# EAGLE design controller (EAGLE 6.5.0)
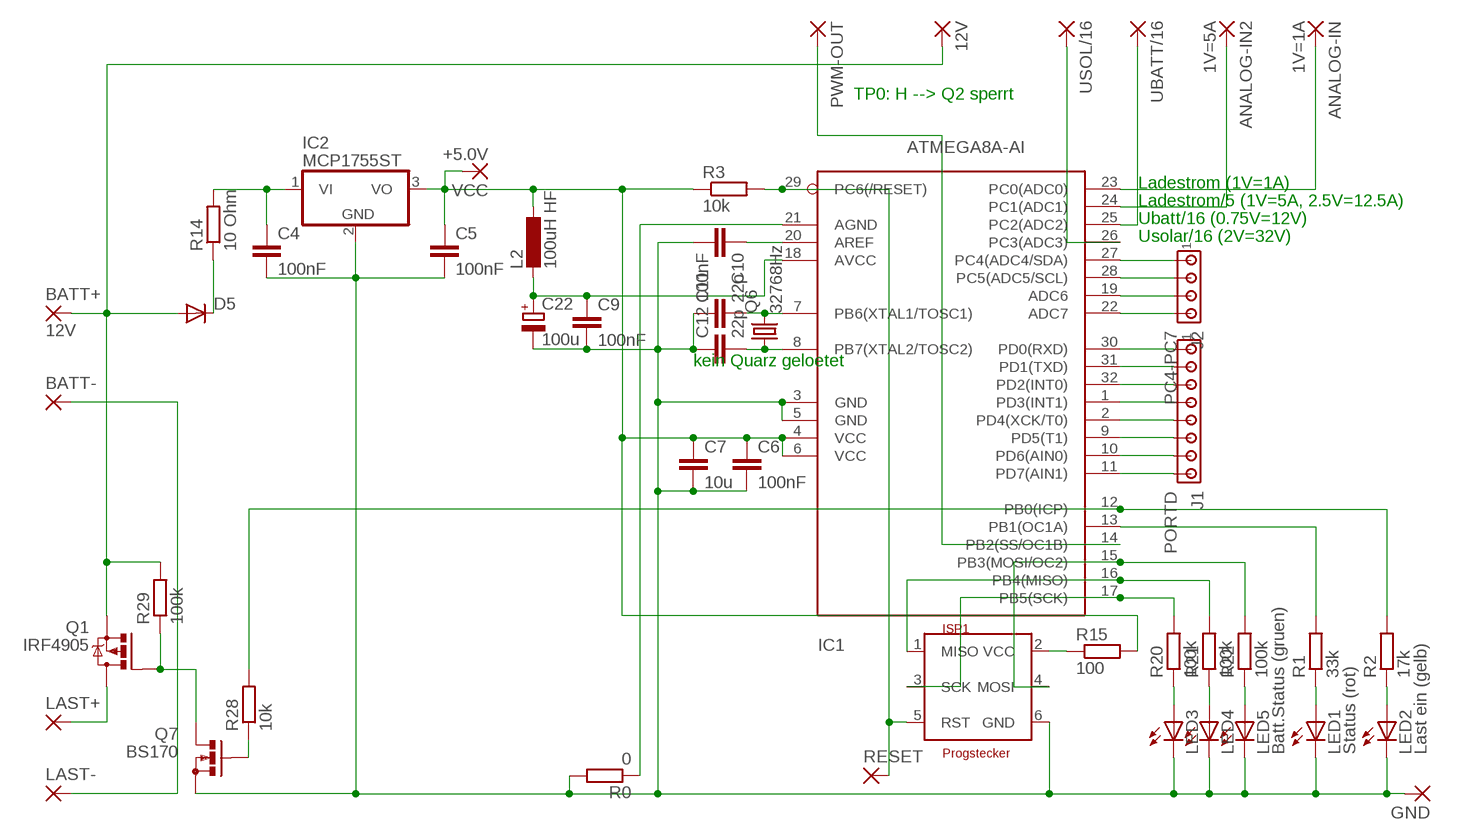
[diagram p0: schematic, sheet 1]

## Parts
12V  WIREPAD2,15/1,0  [2,15/1,0]
ANALOG-IN  1V=1A  WIREPAD2,15/1,0  [2,15/1,0]
ANALOG-IN2  1V=5A  WIREPAD2,15/1,0  [2,15/1,0]
BATT+  12V  WIREPAD3,81/1,1  [3,81/1,1]
BATT-  WIREPAD3,81/1,1  [3,81/1,1]
C4  100nF  C-EUC1206  [C1206]
C5  100nF  C-EUC1206  [C1206]
C6  100nF  C-EUC1206K  [C1206K]
C7  10u  C-EUC1206  [C1206]
C9  100nF  C-EUC1206K  [C1206K]
C10  100nF  C-EUC1206K  [C1206K]
C11  22p  C-EU025-024X044  [C025-024X044]
C12  22p  C-EU025-024X044  [C025-024X044]
C22  100u  CPOL-EUE2.5-5  [E2,5-5]
D5  1N4004  [DO41-10]
GND  WIREPAD2,15/1,0  [2,15/1,0]
IC1  ATMEGA8A-AI  MEGA8-AI  [TQFP32-08]
IC2  MCP1755ST  MCP1703DB  [SOT223]
ISP1  Progstecker  ISP6N  [ISP6]
J1  PORTD  MTA08-100  [10X08MTA]
J2  PC4-PC7  MTA04-100  [10X04MTA]
L2  100uH HF  L-EU0204/7  [0204/7]
LAST+  WIREPAD3,81/1,1  [3,81/1,1]
LAST-  WIREPAD3,81/1,1  [3,81/1,1]
LED1  Status (rot)  LEDSFH482  [SFH482]
LED2  Last ein (gelb)  LEDSFH482  [SFH482]
LED3  LEDSFH482  [SFH482]
LED4  LEDSFH482  [SFH482]
LED5  Batt.Status (gruen)  LEDSFH482  [SFH482]
PWM-OUT  WIREPAD2,15/1,0  [2,15/1,0]
Q1  IRF4905  IRF9530  [TO220BV]
Q6  32768Hz  CRYSTALTC26V  [TC26V]
Q7  BS170  [SOT54E]
R0  0  R-EU_R1206  [R1206]
R1  33k  R-EU_0204/2V  [0204V@1]
R2  17k  R-EU_0204/2V  [0204V@1]
R3  10k  R-EU_M1406  [M1406]
R14  10 Ohm  R-EU_0204/5  [0204/5@1]
R15  100  R-EU_0204/5  [0204/5@1]
R20  100k  R-EU_0204/2V  [0204V@1]
R21  100k  R-EU_0204/2V  [0204V@1]
R22  100k  R-EU_0204/2V  [0204V@1]
R28  10k  R-EU_0204/7  [0204/7@1]
R29  100k  R-EU_0204/5  [0204/5@1]
RESET  WIREPAD1,6/0,8  [1,6/0,8]
UBATT/16  WIREPAD2,15/1,0  [2,15/1,0]
USOL/16  WIREPAD2,15/1,0  [2,15/1,0]
VCC  +5.0V  WIREPAD2,54/0,9  [2,54/0,9]

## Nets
AGND [duenn]: IC1.21(AGND) R0.1
AVCC [duenn]: C9.1 C22.+ IC1.18(AVCC) L2.2
GND [dick]: C4.2 C5.2 C6.2 C7.2 C9.2 C10.2 C11.1 C12.1 C22.- GND.1(P) IC1.3(GND) IC1.5(GND) IC2.2(GND) ISP1.6(GND) LED1.K(C) LED2.K(C) LED3.K(C) LED4.K(C) LED5.K(C) Q7.S R0.2
N$1 [dick]: LED1.A R1.1
N$2: IC1.12(PB0(ICP)) R2.2 R28.2
N$3: IC1.17(PB5(SCK)) ISP1.3(SCK) R20.2
N$4: IC1.13(PB1(OC1A)) R1.2
N$5 [dick]: LED2.A R2.1
N$6 [duenn]: IC1.26(PC3(ADC3)) USOL/16.1(P)
N$7: IC1.14(PB2(SS/OC1B)) PWM-OUT.1(P)
N$8 [dick]: Q7.G R28.1
N$9 [duenn]: IC1.25(PC2(ADC2)) UBATT/16.1(P)
N$10: C10.1 IC1.20(AREF)
N$11: ISP1.2(VCC) R15.1
N$12 [duenn]: ANALOG-IN2.1(P) IC1.24(PC1(ADC1))
N$13 [duenn]: ANALOG-IN.1(P) IC1.23(PC0(ADC0))
N$14 [dick]: D5.C R14.1
N$15: IC1.27(PC4(ADC4/SDA)) J2.1
N$16: IC1.28(PC5(ADC5/SCL)) J2.2
N$17: IC1.19(ADC6) J2.3
N$18 [dick]: C4.1 IC2.1(VI) R14.2
N$19: IC1.22(ADC7) J2.4
N$25: IC1.16(PB4(MISO)) ISP1.1(MISO) R21.2
N$26: IC1.29(PC6(/RESET)) ISP1.5(RST) R3.2 RESET.1(P)
N$27: IC1.15(PB3(MOSI/OC2)) ISP1.4(MOSI) R22.2
N$31 [dick]: LED3.A R20.1
N$33 [dick]: LED4.A R21.1
N$34 [dick]: LED5.A R22.1
N$35: C11.2 IC1.7(PB6(XTAL1/TOSC1)) Q6.2
N$36: C12.2 IC1.8(PB7(XTAL2/TOSC2)) Q6.1
N$43 [sehrdick]: LAST+.1(P) Q1.D
N$44 [sehrdick]: 12V.1(P) BATT+.1(P) D5.A Q1.S R29.2
N$45 [dick]: Q1.G Q7.D R29.1
N$46 [sehrdick]: BATT-.1(P) LAST-.1(P)
N$50: IC1.30(PD0(RXD)) J1.1
N$51: IC1.31(PD1(TXD)) J1.2
N$52: IC1.32(PD2(INT0)) J1.3
N$53: IC1.1(PD3(INT1)) J1.4
N$54: IC1.2(PD4(XCK/T0)) J1.5
N$55: IC1.9(PD5(T1)) J1.6
N$56: IC1.10(PD6(AIN0)) J1.7
N$57: IC1.11(PD7(AIN1)) J1.8
VCC [duenn]: C5.1 C6.1 C7.1 IC1.4(VCC) IC1.6(VCC) IC2.3(VO) L2.1 R3.1 R15.2 VCC.1(P)

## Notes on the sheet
- TP0: H --> Q2 sperrt
- Ladestrom (1V=1A)
- Ladestrom/5 (1V=5A, 2.5V=12.5A)
- Ubatt/16 (0.75V=12V)
- Usolar/16 (2V=32V)
- kein Quarz geloetet

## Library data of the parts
12V ANALOG-IN ANALOG-IN2 BATT+ BATT- GND LAST+ LAST- PWM-OUT RESET UBATT/16 USOL/16 VCC = wirepad:WIREPAD: Wire PAD connect wire on PCB
C4-C7 C9-C12 = rcl:C-EU: CAPACITOR, European symbol
C22 = rcl:CPOL-EU: POLARIZED CAPACITOR, European symbol
D5 = diode:1N4004: DIODE
IC1 = avr-7:MEGA8: MICROCONTROLLER 8 Kbytes FLASH 1 kbytes SRAM 512 bytes EEPROM USART 6-channel 10 bit ADC 2-channel 8 bit ADC
IC2 = linear:MCP1703: 250 mA, 16V, Low Quiescent Current LDO Regulator Source: http://ww1.microchip.com/downloads/en/DeviceDoc/22049b.pdf
ISP1 = stecker:ISP6: ISP-Stecker 6polig
J1 = con-amp:MTA08-100: AMP connector
J2 = con-amp:MTA04-100: AMP connector
L2 = rcl:L-EU: INDUCTOR, European symbol
LED1-LED5 = led:LED: LED
Q1 = transistor-power:IRF9530: P-CHANNEL HEXFET POWER-MOS-FET Source: http://www.irf.com/product-info/datasheets/data/irf9530.pdf
Q6 = crystal:CRYSTAL: CRYSTAL; OC_FARNELL: unknown; OC_NEWARK: unknown
Q7 = transistor-small-signal:BS170: N-CHANNEL MOS FET
R0 R1-R3 R14 R15 R20-R22 R28 R29 = rcl:R-EU_: RESISTOR, European symbol

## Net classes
1 dick: width 0.508 mm, clearance 0.203 mm
2 sehrdick: width 2.032 mm, clearance 0.508 mm
3 duenn: width 0.381 mm

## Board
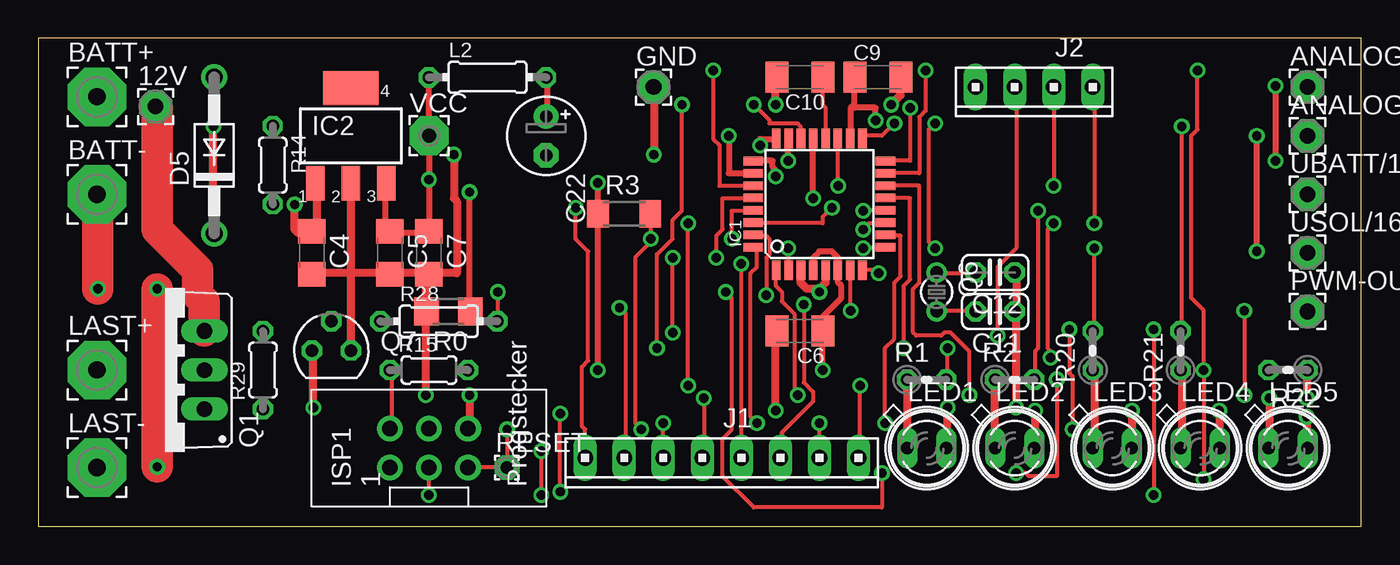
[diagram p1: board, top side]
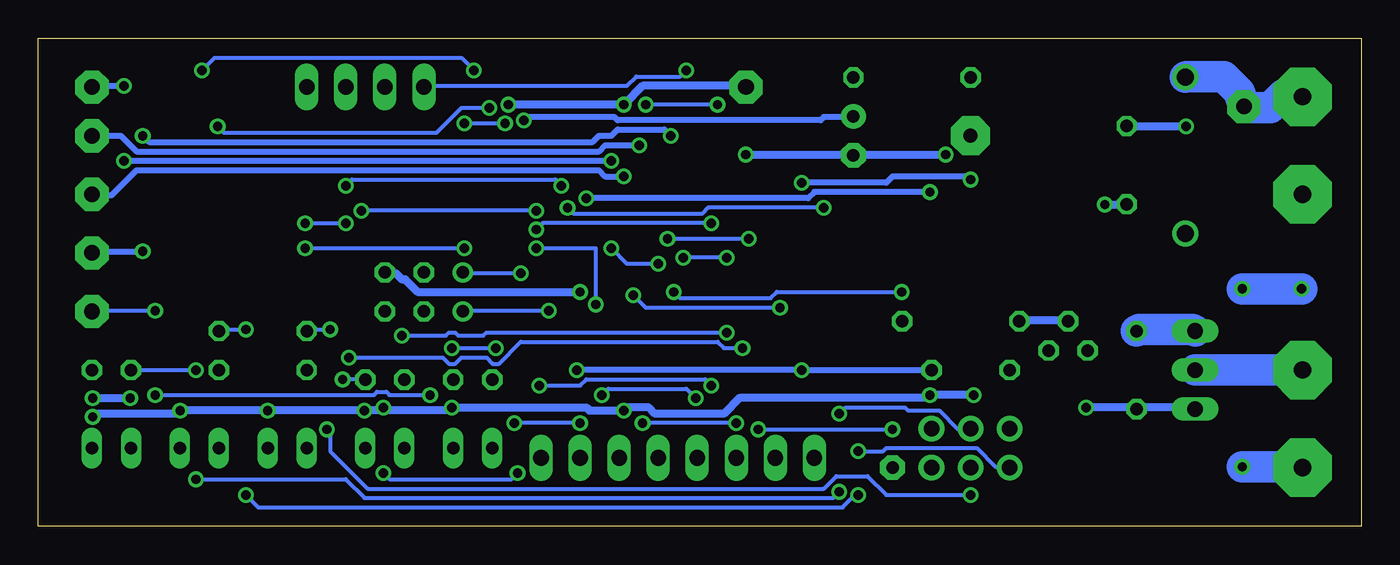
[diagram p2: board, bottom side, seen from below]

Size 86.03 x 31.74 mm. Coordinates in mm from the lower left corner, seen from the top.
Outline: 0,0 86.03,0 86.03,31.74 0,31.74 0,0
Copper layers (1*16): Top 0.035mm / dielectric 1.5mm / Bottom 0.035mm
Design rules "default": minimum track width 10mil, minimum drill 24mil, track to track 8mil, track to pad 8mil, pad to pad 8mil, via to via 8mil, smd to smd 8mil, copper to edge 40mil, drill to drill 8mil, minimum pad ring 10mil, minimum via ring 8mil, stop-mask expansion 4mil, vias tented up to drill 0mil, thermal gap 10mil

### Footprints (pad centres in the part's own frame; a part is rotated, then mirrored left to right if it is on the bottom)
2,15/1,0 = drill 1.016 pad 2.159 octagon: 1 0,0
3,81/1,1 = drill 1.118 pad 3.81 octagon: 1 0,0
C1206 = smd 1.6 x 1.8: 1 -1.4,0; 2 1.4,0
C1206K = smd 1.5 x 2: 1 -1.5,0; 2 1.5,0
C025-024X044 = drill 0.813 octagon: 1 -1.27,0; 2 1.27,0
E2,5-5 = drill 0.813 pad 1.6: + -1.27,0 | drill 0.813 pad 1.6 octagon: - 1.27,0
DO41-10 = drill 1.118: A 5.08,0; C -5.08,0
TQFP32-08 = smd 1.27 x 0.559: 1 -4.293,2.8; 2 -4.293,2; 3 -4.293,1.2; 4 -4.293,0.4; 5 -4.293,-0.4; 6 -4.293,-1.2; 7 -4.293,-2; 8 -4.293,-2.8; 17 4.293,-2.8; 18 4.293,-2; 19 4.293,-1.2; 20 4.293,-0.4; 21 4.293,0.4; 22 4.293,1.2; 23 4.293,2; 24 4.293,2.8 | smd 0.559 x 1.27: 9 -2.8,-4.293; 10 -2,-4.293; 11 -1.2,-4.293; 12 -0.4,-4.293; 13 0.4,-4.293; 14 1.2,-4.293; 15 2,-4.293; 16 2.8,-4.293; 25 2.8,4.293; 26 2,4.293; 27 1.2,4.293; 28 0.4,4.293; 29 -0.4,4.293; 30 -1.2,4.293; 31 -2,4.293; 32 -2.8,4.293
SOT223 = smd 1.219 x 2.235: 1 -2.311,-3.099; 2 0,-3.099; 3 2.311,-3.099 | smd 3.6 x 2.2: 4 0,3.099
ISP6 = drill 1 pad 1.676: 1 -1.27,2.54; 2 1.27,2.54; 3 -1.27,0; 4 1.27,0; 5 -1.27,-2.54; 6 1.27,-2.54
10X08MTA = drill 1.016 long: 1 8.89,0; 2 6.35,0; 3 3.81,0; 4 1.27,0; 5 -1.27,0; 6 -3.81,0; 7 -6.35,0; 8 -8.89,0
10X04MTA = drill 1.016 long: 1 3.81,0; 2 1.27,0; 3 -1.27,0; 4 -3.81,0
0204/7 = drill 0.813 octagon: 1 -3.81,0; 2 3.81,0
SFH482 = drill 0.813 long: A -1.27,0; K 1.27,0
TO220BV = drill 1.016 long: D 0,-2.54; G -2.54,-2.54; S 2.54,-2.54
TC26V = drill 0.813: 1 -1.27,0; 2 1.27,0
SOT54E = drill 0.813 octagon: D -1.27,0; G 0,1.905; S 1.27,0
R1206 = smd 1.6 x 1.803: 1 -1.422,0; 2 1.422,0
0204V@1 = drill 0.813 octagon: 1 -1.27,0; 2 1.27,0
M1406 = smd 1.4 x 1.8: 1 -1.7,0; 2 1.7,0
0204/5@1 = drill 0.813 octagon: 1 -2.54,0; 2 2.54,0
0204/7@1 = drill 0.813 octagon: 1 -3.81,0; 2 3.81,0
1,6/0,8 = drill 0.813 pad 1.6 octagon: 1 0,0
2,54/0,9 = drill 0.914 pad 2.54 octagon: 1 0,0

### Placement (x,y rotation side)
12V  7.62,27.3 0 top
ANALOG-IN  82.55,28.57 0 top
ANALOG-IN2  82.55,25.4 0 top
BATT+  3.81,27.94 0 top
BATT-  3.81,21.59 0 top
C4  17.78,17.78 270 top
C5  22.86,17.78 270 top
C6  49.53,12.7 180 top
C7  25.4,17.78 270 top
C9  54.61,29.21 0 top
C10  49.53,29.21 180 top
C11  62.23,13.97 180 top
C12  62.23,16.51 180 top
C22  33.02,25.4 270 top
D5  11.43,24.13 90 top
GND  40.01,28.57 0 top
IC1  50.8,20.95 90 top
IC2  20.32,25.4 0 top
ISP1  25.4,5.08 90 top
J1  44.45,4.45 180 top
J2  64.77,28.57 180 top
L2  29.21,29.21 0 top
LAST+  3.81,10.16 0 top
LAST-  3.81,3.81 0 top
LED1  57.78,5.08 0 top
LED2  63.5,5.08 0 top
LED3  69.85,5.08 0 top
LED4  75.56,5.08 0 top
LED5  81.28,5.08 0 top
PWM-OUT  82.55,13.97 0 top
Q1  8.26,10.16 90 top
Q6  58.42,15.24 270 top
Q7  19.05,11.43 0 top
R0  26.67,13.97 180 top
R1  57.78,9.53 0 top
R2  63.5,9.53 0 top
R3  38.1,20.32 0 top
R14  15.24,23.5 270 top
R15  25.4,10.16 0 top
R20  68.58,11.43 90 top
R21  74.3,11.43 90 top
R22  81.28,10.16 180 top
R28  26.04,13.34 0 top
R29  14.61,10.16 90 top
RESET  30.48,3.81 0 top
UBATT/16  82.55,21.59 0 top
USOL/16  82.55,17.78 0 top
VCC  25.4,25.4 0 top

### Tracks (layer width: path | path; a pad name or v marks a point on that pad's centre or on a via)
AGND  (via drill 0.61)
  Top 0.381: v50.39,21.34 50.39,25.2 IC1.21 | v28.04,21.74 28.04,14.02 R0.1
  Bottom 0.381: v50.39,21.34 35.97,21.34 35.56,21.74 v28.04,21.74
AVCC  (via drill 0.61)
  Top 0.381: 52.93,27.33 53.03,27.43 53.03,29.06 C9.1 | 52.93,27.33 52.83,27.23 52.83,25.4 IC1.18 | L2.2 33.12,29.06 33.12,26.82 C22.+ | v54.46,26.42 54.46,27.23 53.03,27.23 52.93,27.33
  Bottom 0.381: v54.46,26.42 54.25,26.62 48.56,26.62 48.36,26.42 35.15,26.42 34.95,26.62 33.12,26.62 C22.+
GND  (via drill 0.61)
  Top 0.508: 50.8,15.44 49.99,15.44 49.58,15.85 49.58,16.66 IC1.3 | 50.8,15.44 51.21,15.85 IC1.5 | v50.8,15.24 50.8,15.44 | C12.1 63.6,16.46 63.6,14.02 C11.1 63.6,13.82 v63.6,7.72 | v47.95,7.52 47.95,12.6 C6.2 | v59.13,7.72 59.13,5.08 LED1.K | v64.82,7.52 64.82,5.08 LED2.K | v71.12,7.52 LED3.K | v76.81,7.52 76.81,5.08 LED4.K | v82.5,7.11 82.5,5.08 LED5.K | 20.32,16.46 17.88,16.46 C4.2 | IC2.2 20.32,16.46 | 20.32,16.46 Q7.S | C7.2 25.4,16.46 22.96,16.46 C5.2 22.76,16.46 20.32,16.46 | C7.2 25.2,16.26 25.2,14.02 R0.2 25.2,13.82 v25.2,8.53 | v28.04,8.53 28.04,6.5 ISP1.6 | v40.03,24.18 40.03,28.45 GND.1 | v47.95,27.43 47.95,29.06 C10.2 | v55.47,27.43 56.08,28.04 56.08,29.06 C9.2 | v27.03,24.18 27.03,21.34 27.23,21.13 27.23,16.46 25.6,16.46 C7.2
  Bottom 0.508: v50.8,15.24 61.37,15.24 62.18,16.05 62.38,16.05 62.79,16.46 63.4,16.46 C12.1 | 63.6,7.52 59.13,7.52 v59.13,7.72 50.39,7.72 50.19,7.52 v47.95,7.52 47.95,7.72 46.33,7.72 45.92,7.32 41.45,7.32 40.44,8.33 28.04,8.33 v28.04,8.53 v25.2,8.53 | 63.6,7.52 v64.82,7.52 v71.12,7.52 v76.81,7.52 76.81,7.32 82.3,7.32 v82.5,7.11 | v63.6,7.72 63.6,7.52 | v40.03,24.18 33.12,24.18 C22.- 32.92,24.18 v27.03,24.18 | GND.1 40.03,28.65 46.74,28.65 v47.95,27.43 v55.47,27.43
N$1
  Top 0.508: LED1.A 56.49,5.08 56.49,9.35 R1.1
N$2  (via drill 0.61)
  Top 0.254: v65.02,20.52 65.02,11.58 64.82,11.38 64.82,9.55 R2.2 | v53.65,20.52 55.07,20.52 IC1.12 | v29.87,15.24 29.87,13.41 R28.2 | v44.7,15.24 45.11,14.83 45.11,6.3 44.5,5.69 44.5,3.25 46.53,1.22 54.86,1.22 v54.86,3.45 | v63.6,3.45 64.21,3.45 64.41,3.25 66.24,3.25 v66.24,9.55
  Bottom 0.254: v53.65,20.52 v65.02,20.52 | v29.87,15.24 38,15.24 38.41,14.83 44.3,14.83 v44.7,15.24 | v54.86,3.45 55.27,3.05 63.2,3.05 v63.6,3.45 | v66.24,9.55 64.82,9.55 R2.2
N$3  (via drill 0.61)
  Top 0.254: v55.68,26.21 54.86,25.4 53.65,25.4 IC1.17 | v58.32,26.21 57.91,25.81 57.91,18.49 v58.32,18.09 | v68.68,18.09 68.68,12.8 R20.2 | v25.4,2.03 ISP1.3 | v67.26,6.3 67.26,9.75 67.06,9.96 v67.06,12.8
  Bottom 0.254: v58.32,26.21 v55.68,26.21 | v68.68,18.09 v58.32,18.09 | v25.4,2.03 30.89,2.03 32.11,3.25 34.14,3.25 34.95,2.44 64.62,2.44 67.06,4.88 67.06,6.3 v67.26,6.3 | v67.06,12.8 68.48,12.8 R20.2
N$4  (via drill 0.61)
  Top 0.254: v56.29,11.58 56.29,15.65 56.69,16.05 56.69,21.34 55.27,21.34 IC1.13 | v59.13,11.58 59.13,9.55 R1.2
  Bottom 0.254: v59.13,11.58 v56.29,11.58
N$5
  Top 0.508: LED2.A 62.18,5.08 62.18,9.35 R2.1
N$6  (via drill 0.61)
  Top 0.381: v44.91,25.4 44.91,22.96 46.33,22.96 IC1.26 | v79.25,17.88 v79.25,25.4
  Bottom 0.381: v44.91,25.4 45.31,25.81 48.36,25.81 48.77,25.4 49.58,25.4 49.99,24.99 78.84,24.99 v79.25,25.4 | v79.25,17.88 82.5,17.88 USOL/16.1
N$7  (via drill 0.61)
  Top 0.254: v60.55,8.53 60.55,11.38 59.33,12.6 58.93,12.6 58.73,12.39 57.1,12.39 56.9,12.6 56.9,15.44 57.3,15.85 57.3,22.15 55.27,22.15 IC1.14 | v78.44,14.02 v78.44,8.53
  Bottom 0.254: v60.55,8.53 63.2,8.53 63.4,8.74 64.01,8.74 64.21,8.53 v78.44,8.53 | v78.44,14.02 82.5,14.02 PWM-OUT.1
N$8
  Bottom 0.508: Q7.G 19.1,13.41 22.15,13.41 R28.1
N$9  (via drill 0.61)
  Top 0.381: v47.95,22.76 47.95,23.16 47.75,23.37 47.75,23.77 46.53,23.77 IC1.25
  Bottom 0.381: v47.95,22.76 49.17,22.76 49.58,23.16 79.65,23.16 81.28,21.54 82.5,21.54 UBATT/16.1
N$10
  Top 0.254: IC1.20 51.21,25.4 51.21,27.23 51,27.43 51,29.06 C10.1
N$11
  Top 0.254: ISP1.2 22.96,6.5 22.96,10.16 R15.1
N$12  (via drill 0.61)
  Top 0.381: v46.94,24.79 46.94,25.2 47.95,25.2 IC1.24
  Bottom 0.381: v46.94,24.79 49.17,24.79 49.58,24.38 79.65,24.38 80.67,25.4 ANALOG-IN2.1
N$13  (via drill 0.61)
  Top 0.381: v48.77,23.77 48.77,25.2 IC1.23 | v80.47,28.65 v80.47,23.77
  Bottom 0.381: v80.47,23.77 v48.77,23.77 | v80.47,28.65 82.5,28.65 ANALOG-IN.1
N$14  (via drill 0.61)
  Top 0.508: v11.38,26.01 11.38,19.1 D5.C
  Bottom 0.508: v11.38,26.01 15.24,26.01 R14.1
N$15  (via drill 0.61)
  Top 0.254: v43.89,29.67 43.89,25.2 44.3,24.79 44.3,22.15 46.33,22.15 IC1.27
  Bottom 0.254: v43.89,29.67 44.3,29.26 47.14,29.26 47.75,28.65 60.96,28.65 J2.1
N$16  (via drill 0.61)
  Top 0.254: v44.09,17.48 44.09,18.9 44.5,19.3 44.5,21.34 46.33,21.34 IC1.28 | v41.25,12.6 v41.25,17.48 | v62.38,12.39 62.38,16.87 63.6,18.09 63.6,28.45 J2.2
  Bottom 0.254: v41.25,17.48 v44.09,17.48 | v41.25,12.6 56.9,12.6 57.1,12.39 58.73,12.39 58.93,12.6 59.33,12.6 59.54,12.39 v62.38,12.39
N$17  (via drill 0.61)
  Top 0.254: v52.02,22.15 52.02,25.2 IC1.19 | J2.3 v66.04,22.15
  Bottom 0.254: v52.02,22.15 52.43,22.55 65.63,22.55 v66.04,22.15
N$18  (via drill 0.61)
  Top 0.508: IC2.1 18.09,22.15 18.09,19.1 17.88,19.1 C4.1 17.68,19.1 16.87,19.1 16.66,19.3 v16.66,20.93
  Bottom 0.508: v16.66,20.93 15.24,20.93 R14.2
N$19  (via drill 0.61)
  Top 0.254: v46.53,27.43 47.55,26.42 47.55,26.21 49.38,26.21 49.58,26.01 49.58,25.4 IC1.22 | v41.86,27.43 41.86,20.52 41.25,19.91 41.25,18.69 40.23,17.68 v40.23,11.58 | v65.84,10.97 65.84,11.38 65.63,11.58 65.63,19.3 v66.04,19.71 | v68.68,19.71 68.68,28.45 J2.4
  Bottom 0.254: v41.86,27.43 v46.53,27.43 | v40.23,11.58 41.45,11.58 41.86,11.99 54.66,11.99 56.08,10.57 56.49,10.57 56.9,10.97 58.52,10.97 58.93,10.57 59.33,10.57 59.74,10.97 v65.84,10.97 | v68.68,19.71 v66.04,19.71
N$25  (via drill 0.61)
  Top 0.254: v56.69,27.23 56.69,23.77 55.27,23.77 IC1.16 | v74.37,26.01 74.37,12.8 R21.2 | v32.72,2.03 v32.72,4.88 | v72.54,12.8 v72.54,2.03
  Bottom 0.254: v56.69,27.23 58.52,27.23 60.15,25.6 73.97,25.6 v74.37,26.01 | v32.72,4.88 31.09,4.88 30.89,5.08 24.99,5.08 23.77,3.86 22.96,3.86 ISP1.1 | v32.72,2.03 32.92,2.03 33.73,1.22 71.73,1.22 v72.54,2.03 | v72.54,12.8 74.17,12.8 R21.2
N$26  (via drill 0.61)
  Top 0.254: 30.48,3.86 28.04,3.86 ISP1.5 | v45.11,18.69 45.11,20.52 46.33,20.52 IC1.29 | R3.2 39.83,20.32 v39.83,18.69 39.83,18.49 38.81,17.48 38.81,6.71 v39.22,6.3 | v30.48,6.3 30.48,3.86 | 30.48,3.86 RESET.1
  Bottom 0.254: v39.83,18.69 v45.11,18.69 | v39.22,6.3 v30.48,6.3
N$27  (via drill 0.61)
  Top 0.254: v57.71,29.67 57.71,27.03 57.3,26.62 57.3,22.96 55.27,22.96 IC1.15 | v75.39,29.67 75.39,25.81 74.98,25.4 74.98,14.83 75.79,14.02 v75.79,10.16 v75.79,3.05 | v33.93,2.23 v33.93,7.32
  Bottom 0.254: v57.71,29.67 58.52,30.48 74.57,30.48 v75.39,29.67 | R22.2 v75.79,10.16 | v33.93,7.32 33.53,7.72 29.67,7.72 29.46,7.52 27.43,7.52 26.21,6.3 25.4,6.3 ISP1.4 | v33.93,2.23 34.34,1.83 64.82,1.83 66.04,3.05 v75.79,3.05
N$31
  Top 0.508: LED3.A 68.68,5.08 68.68,10.16 R20.1
N$33
  Top 0.508: LED4.A 74.37,5.08 74.37,10.16 R21.1
N$34  (via drill 0.61)
  Top 0.508: v80.06,8.33 80.06,5.08 LED5.A | v82.5,8.33 82.5,10.16 R22.1
  Bottom 0.508: v82.5,8.33 v80.06,8.33
N$35  (via drill 0.61)
  Top 0.254: C11.2 60.96,14.02 58.52,14.02 Q6.2 | v52.83,14.02 52.83,16.66 IC1.7
  Bottom 0.254: v52.83,14.02 58.32,14.02 Q6.2
N$36  (via drill 0.61)
  Top 0.254: C12.2 60.96,16.46 58.52,16.46 Q6.1 | IC1.8 54.66,16.66 v54.66,16.46
  Bottom 0.254: v54.66,16.46 58.32,16.46 Q6.1
N$43
  Bottom 2.032: Q1.D LAST+.1
N$44
  Top 2.032: Q1.S 10.77,12.8 10.77,14.63 10.36,15.04 10.36,16.66 7.72,19.3 7.72,27.23 12V.1
  Bottom 2.032: R29.2 14.43,12.8 10.97,12.8 Q1.S | BATT+.1 3.86,28.04 5.08,28.04 5.89,27.23 7.52,27.23 12V.1 7.92,28.25 8.94,29.26 11.38,29.26 D5.A
N$45  (via drill 0.61)
  Top 0.508: v17.88,7.72 17.88,11.38 Q7.D
  Bottom 0.508: Q1.G 10.97,7.72 14.43,7.72 R29.1 14.83,7.72 v17.88,7.72
N$46  (via drill 0.61)
  Top 2.032: v7.72,15.44 v7.72,3.86 | v3.86,15.44 3.86,21.54 BATT-.1
  Bottom 2.032: v7.72,3.86 3.86,3.86 LAST-.1 | v3.86,15.44 v7.72,15.44
N$50  (via drill 0.61)
  Top 0.254: v51.61,20.73 51,20.12 51,19.71 46.53,19.71 IC1.30 | v34.95,20.73 34.95,18.69 35.76,17.88 35.76,10.77 35.36,10.36 35.36,6.5 35.56,6.3 J1.1
  Bottom 0.254: v51.61,20.73 51.21,20.32 42.88,20.32 42.47,20.73 v34.95,20.73
N$51  (via drill 0.61)
  Top 0.254: v37.8,14.22 38.2,13.82 38.2,4.47 J1.2 | v47.35,15.04 47.35,17.48 47.55,17.68 47.55,18.69 47.35,18.9 46.53,18.9 IC1.31
  Bottom 0.254: v37.8,14.22 46.53,14.22 v47.35,15.04
N$52  (via drill 0.61)
  Top 0.254: v46.74,6.71 46.33,7.11 46.33,16.46 46.74,16.87 46.74,18.09 46.53,18.09 IC1.32 | J1.3 v40.64,6.71
  Bottom 0.254: v40.64,6.71 v46.74,6.71
N$53  (via drill 0.61)
  Top 0.254: v43.28,8.33 43.28,4.47 J1.4 | v49.38,8.53 49.17,8.74 49.17,13.82 48.36,14.63 48.36,15.24 47.95,15.65 47.95,16.66 IC1.1
  Bottom 0.254: v43.28,8.33 43.89,8.94 48.97,8.94 v49.38,8.53
N$54  (via drill 0.61)
  Top 0.254: v48.77,18.09 48.77,16.66 IC1.2 | J1.5 v45.72,17.07
  Bottom 0.254: v48.77,18.09 47.75,17.07 v45.72,17.07
N$55  (via drill 0.61)
  Top 0.254: v49.78,14.43 49.78,9.35 50.39,8.74 50.39,8.13 48.36,6.1 48.36,4.47 J1.6 | v53.65,18.09 55.07,18.09 IC1.9
  Bottom 0.254: v49.78,14.43 49.78,18.09 v53.65,18.09
N$56  (via drill 0.61)
  Top 0.254: v55.07,6.71 55.07,11.58 55.68,12.19 55.68,15.85 56.08,16.26 56.08,18.9 55.27,18.9 IC1.10 | J1.7 v50.8,6.71
  Bottom 0.254: v50.8,6.71 v55.07,6.71
N$57  (via drill 0.61)
  Top 0.254: v53.65,19.3 54.05,19.71 55.07,19.71 IC1.11 | v42.27,9.14 v42.27,19.71 | v53.44,9.14 53.44,4.47 J1.8
  Bottom 0.254: v53.65,19.3 53.24,19.71 v42.27,19.71 | v42.27,9.14 42.67,9.55 50.39,9.55 50.8,9.14 v53.44,9.14
VCC  (via drill 0.61)
  Top 0.381: IC2.3 22.55,22.15 22.55,19.1 22.76,19.1 C5.1 22.96,19.1 25.4,19.1 C7.1 v25.4,22.55 VCC.1 L2.1 | 52.02,16.66 52.02,17.48 51.61,17.88 50.8,17.88 50.39,17.48 IC1.4 | 52.02,16.66 52.02,15.85 52.22,15.65 52.22,14.83 51,13.61 51,12.8 C6.1 51,12.6 v51,10.16 | 52.02,16.66 IC1.6 | v36.37,22.35 36.37,20.32 | 36.37,20.32 v36.37,10.16 | 36.37,20.32 R3.1
  Bottom 0.381: v36.37,22.35 30.89,22.35 30.48,22.76 25.6,22.76 v25.4,22.55 | R15.2 v36.37,10.16 v51,10.16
